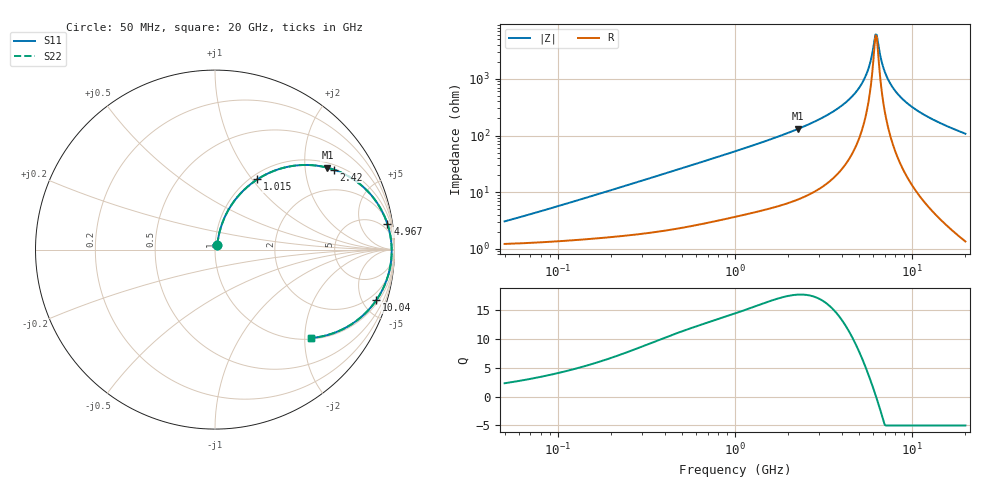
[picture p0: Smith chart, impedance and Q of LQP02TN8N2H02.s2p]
!Murata Part Number: LQP02TN8N2H02
!These Parameters are Measured in Series Mode Connection
!  o--[Z]--o
!Port1  Port2
!  o-------o
!Freq. Start=50[MHz] Stop=20[GHz], 401[Steps]
# Hz S RI R 50
!Freq.(Hz) S11(Real) S11(Imag) S21(Real) S21(Imag) S12(Real) S12(Imag) S22(Real) S22(Imag)
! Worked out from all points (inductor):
!   401 points, 50 MHz to 20 GHz, reference 50 ohm
!   read as one part in series: L = 8.76 nH near 68.48 MHz
!   highest Q = 17.6 at 2.279 GHz (marker M1), where L = 9.16 nH
!   self-resonance near 6.218 GHz
!   S11 on the Smith chart (normalised r, x): 50 MHz: 1.02, +0.06; 1.015 GHz: 1.07, +1.06; 2.42 GHz: 1.16, +2.84; 4.967 GHz: 3, +13; 10.04 GHz: 1.26, -6.31; 20 GHz: 1.03, -2.15
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5e7  0.0127 0.0272  0.9873 -0.0272  0.9873 -0.0272  0.0127 0.0272
1.364002e8  0.0195 0.0715  0.9805 -0.0715  0.9805 -0.0715  0.0195 0.0715
3.721004e8  0.0547 0.182  0.9453 -0.182  0.9453 -0.182  0.0547 0.182
1e9  0.2314 0.3884  0.7686 -0.3884  0.7686 -0.3884  0.2314 0.3884
1.015091e9  0.2364 0.3916  0.7636 -0.3916  0.7636 -0.3916  0.2364 0.3916
1.590961e9  0.4281 0.4655  0.5719 -0.4655  0.5719 -0.4655  0.4281 0.4655
2.279204e9  0.6265 0.4562  0.3735 -0.4562  0.3735 -0.4562  0.6265 0.4562
2.419936e9  0.6605 0.446  0.3395 -0.446  0.3395 -0.446  0.6605 0.446
2.728004e9  0.7269 0.4177  0.2731 -0.4177  0.2731 -0.4177  0.7269 0.4177
3.908127e9  0.8937 0.274  0.1063 -0.274  0.1063 -0.274  0.8937 0.274
4.966507e9  0.961 0.1415  0.039 -0.1415  0.039 -0.1415  0.961 0.1415
5.598765e9  0.9784 0.069  0.0216 -0.069  0.0216 -0.069  0.9784 0.069
5.856089e9  0.9821 0.0413  0.0179 -0.0413  0.0179 -0.0413  0.9821 0.0413
6.125241e9  0.984 0.0133  0.016 -0.0133  0.016 -0.0133  0.984 0.0133
6.217679e9  0.9844 0.00398  0.0156 -0.00398  0.0156 -0.00398  0.9844 0.00398
6.406762e9  0.9844 -0.0147  0.0156 0.0147  0.0156 0.0147  0.9844 -0.0147
6.905011e9  0.9814 -0.0614  0.0186 0.0614  0.0186 0.0614  0.9814 -0.0614
7.442007e9  0.9738 -0.1077  0.0262 0.1077  0.0262 0.1077  0.9738 -0.1077
8.389408e9  0.9524 -0.18  0.0476 0.18  0.0476 0.18  0.9524 -0.18
1.004137e10  0.8995 -0.2808  0.1005 0.2808  0.1005 0.2808  0.8995 -0.2808
1.354865e10  0.7634 -0.4141  0.2366 0.4141  0.2366 0.4141  0.7634 -0.4141
2e10  0.536 -0.4925  0.464 0.4925  0.464 0.4925  0.536 -0.4925
